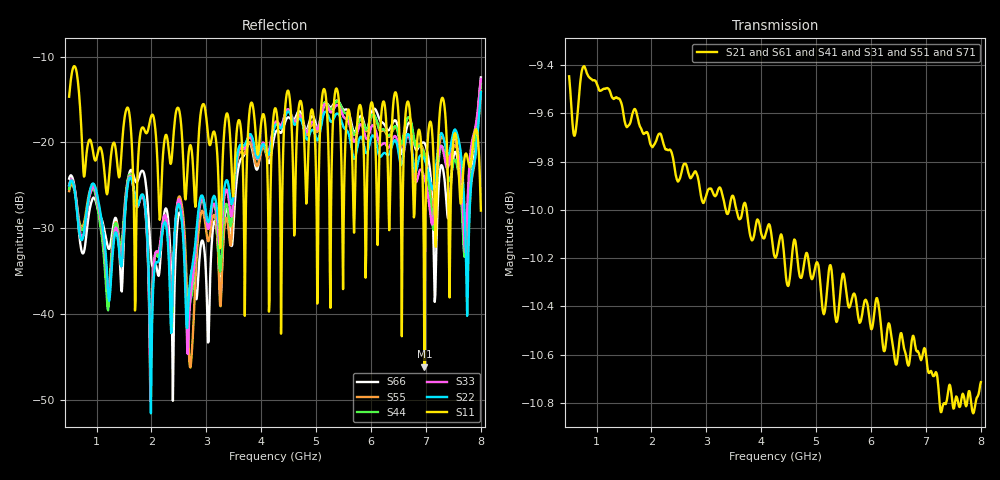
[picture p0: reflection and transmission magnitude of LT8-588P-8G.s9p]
! MTS Systemtechnik GmbH
! S-Parameters
! Model: LT8-588P-8G
! Rohde & Schwarz ZVB8 2Ports - Version 3.20 - 1145.1010k08 SN: 100119
! Converted & adapted with Octave
!		|  MTS  |
!		|  |--o OUT 8 (Port 9)
!		|  |--o OUT 7 (Port 8)
!		|  |--o OUT 6 (Port 7)
!		|  |--o OUT 5 (Port 6)
! C (Port 1) o--| LT8-588P-8G |
!		|  |--o OUT 4 (Port 5)
!		|  |--o OUT 3 (Port 4)
!		|  |--o OUT 2 (Port 3)
!		|  |--o OUT 1 (Port 2)
! S9P File: Measurements:
! <S11,S12,S13,S14,S15,S16,S17,S18,S19>,
! <S21,S22,S23,S24,S25,S26,S27,S28,S29>,
! <S31,S32,S33,S34,S35,S36,S37,S38,S39>,
! <S41,S42,S43,S44,S45,S46,S47,S48,S49>,
! <S51,S52,S53,S54,S55,S56,S57,S58,S59>,
! <S61,S62,S63,S64,S65,S66,S67,S68,S69>,
! <S71,S72,S73,S74,S75,S76,S77,S78,S79>,
! <S81,S82,S83,S84,S85,S86,S87,S88,S89>,
! <S91,S92,S93,S94,S95,S96,S97,S98,S99>:
# HZ  S  DB  R  50.00
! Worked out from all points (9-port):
!   751 points, 500 MHz to 8 GHz, reference 50 ohm
!   strongest paths, dB at 500 MHz, 2.37 GHz, 4.25 GHz, 6.13 GHz, 8 GHz:
!     S21: -9.4, -9.8, -10.2, -10.4, -10.7
!     S61: -9.4, -9.8, -10.2, -10.5, -10.9
!     S41: -9.4, -9.8, -10.2, -10.5, -10.9
!     S31: -9.5, -9.8, -10.3, -10.5, -10.9
!     S51: -9.4, -9.8, -10.3, -10.5, -10.8
!     S71: -9.4, -9.8, -10.2, -10.6, -10.9
!   lowest |S11| = -46.1 dB at 6.97 GHz (marker M1), VSWR 1.01, Z = 49.5 - j0.155 ohm
!   |S11| at or under -10 dB: start of sweep to end of sweep
